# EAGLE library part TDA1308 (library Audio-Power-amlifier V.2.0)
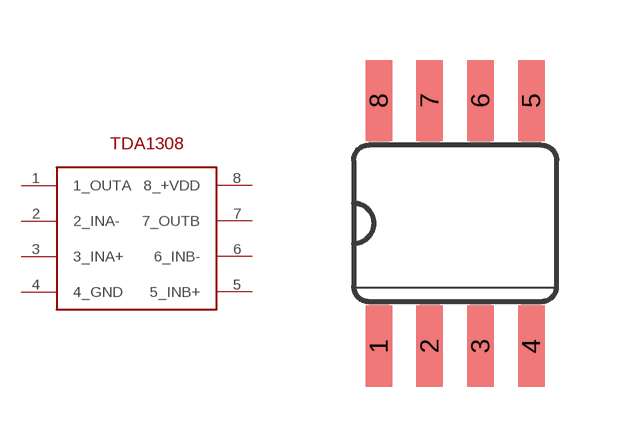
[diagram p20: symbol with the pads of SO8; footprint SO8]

Designator prefix -

## TDA1308SO8  [SO8]
1  1_OUTA
2  2_INA-
3  3_INA+
4  4_GND
5  5_INB+
6  6_INB-
7  7_OUTB
8  8_+VDD

## Footprint SO8 (pad centres in mm)
smd 0.66 x 2.032: 1 -1.905,-3.073; 2 -0.635,-3.073; 3 0.635,-3.073; 4 1.905,-3.073; 5 1.905,3.073; 6 0.635,3.073; 7 -0.635,3.073; 8 -1.905,3.073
